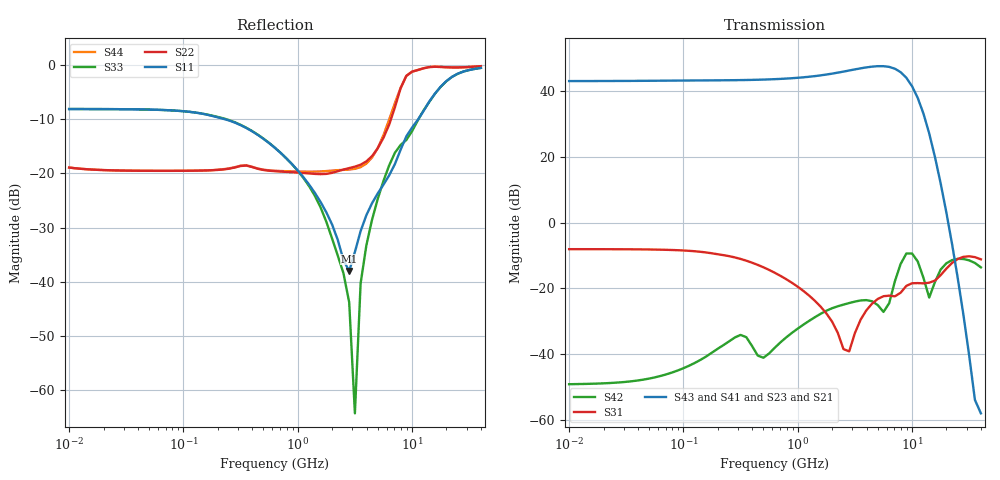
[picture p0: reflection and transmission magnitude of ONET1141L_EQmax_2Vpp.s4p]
! Touchstone Ver. 1.0
! Fri Mar 23 19:25:35 2012
! Number of ports is 4
# Hz	S	DB	R	50.000000
! SCATTERING PARAMETERS  :
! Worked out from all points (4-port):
!   73 points, 10 MHz to 40 GHz, reference 50 ohm
!   strongest paths, dB at 10 MHz, 79.43 MHz, 631 MHz, 5.012 GHz, 40 GHz:
!     S43: 43.0, 43.2, 43.6, 47.6, -58.0
!     S41: 43.0, 43.2, 43.6, 47.6, -58.0
!     S23: 43.0, 43.2, 43.6, 47.5, -58.2
!     S21: 43.0, 43.2, 43.6, 47.6, -58.0
!     S31: -8.1, -8.3, -15.3, -23.2, -11.2
!     S42: -49.1, -45.6, -38.0, -25.1, -13.6
!   lowest |S11| = -38.0 dB at 2.818 GHz (marker M1), VSWR 1.03, Z = 48.8 + j0.225 ohm
!   |S11| at or under -10 dB: 229 MHz to 11.33 GHz (11.1 GHz wide, 192 % of centre)
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1e7  -8.13 -2.0  -109.36 92.2  -8.07 -1.7  -108.83 92.7
     43.02 -177.4  -18.93 24.6  43.02 2.6  -49.47 12.9
     -8.07 -1.7  -109.14 92.1  -8.13 -2.0  -109.00 93.7
     43.03 2.6  -49.13 12.7  43.03 -177.4  -18.92 24.6
2.818383e9  -38.04 169.4  -43.86 -5.7  -44.46 -19.3  -43.86 -5.7
            46.25 79.9  -19.03 -62.0  46.23 -100.3  -23.74 35.2
            -39.14 147.6  -43.84 -5.7  -43.80 -67.4  -43.84 -5.7
            46.26 -99.9  -24.45 39.1  46.25 79.9  -19.30 -64.9
4.466836e9  -25.51 85.7  -45.77 -34.3  -28.08 87.3  -45.76 -34.5
            47.42 4.4  -16.81 -123.7  47.39 -175.7  -25.23 7.4
            -24.63 73.4  -45.76 -34.4  -28.55 107.6  -45.77 -34.2
            47.44 -175.2  -23.90 5.0  47.42 4.6  -17.07 -120.2
6.309573e9  -20.36 75.9  -45.13 -52.2  -20.65 69.3  -45.12 -52.5
            47.33 -86.8  -11.01 178.3  47.28 93.0  -30.79 -113.0
            -22.19 51.6  -45.12 -51.9  -18.52 86.4  -45.13 -51.6
            47.37 93.7  -24.49 -138.8  47.35 -86.4  -10.05 -179.3
8.912509e9  -13.17 60.1  -42.74 -106.3  -20.26 42.4  -42.68 -106.6
            43.93 139.3  -1.99 98.5  43.84 -40.9  -9.36 89.3
            -19.23 56.9  -42.56 -106.4  -13.84 53.6  -42.59 -106.1
            44.04 -40.5  -9.40 86.9  44.04 139.5  -2.04 97.4
1.122018e10  -10.13 38.2  -46.09 -153.0  -18.47 48.4  -45.94 -153.6
             37.83 26.2  -0.94 43.6  37.72 -154.0  -11.96 15.4
             -18.38 43.6  -45.84 -153.6  -10.24 40.2  -45.90 -153.2
             37.89 -154.0  -11.82 15.0  37.88 26.1  -0.92 43.3
4e10  -0.54 -107.5  -58.81 2.2  -11.16 -16.6  -58.55 1.3
      -58.01 34.1  -0.22 -118.6  -58.16 -5.8  -13.60 -28.1
      -11.16 -16.6  -58.64 1.6  -0.54 -107.4  -58.66 1.9
      -58.04 -6.3  -13.60 -28.1  -57.98 33.3  -0.22 -118.6
